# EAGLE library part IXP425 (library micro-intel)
Intel XScale® Core Source: ftp://download.intel.com/design/network/datashts/25247904.pdf
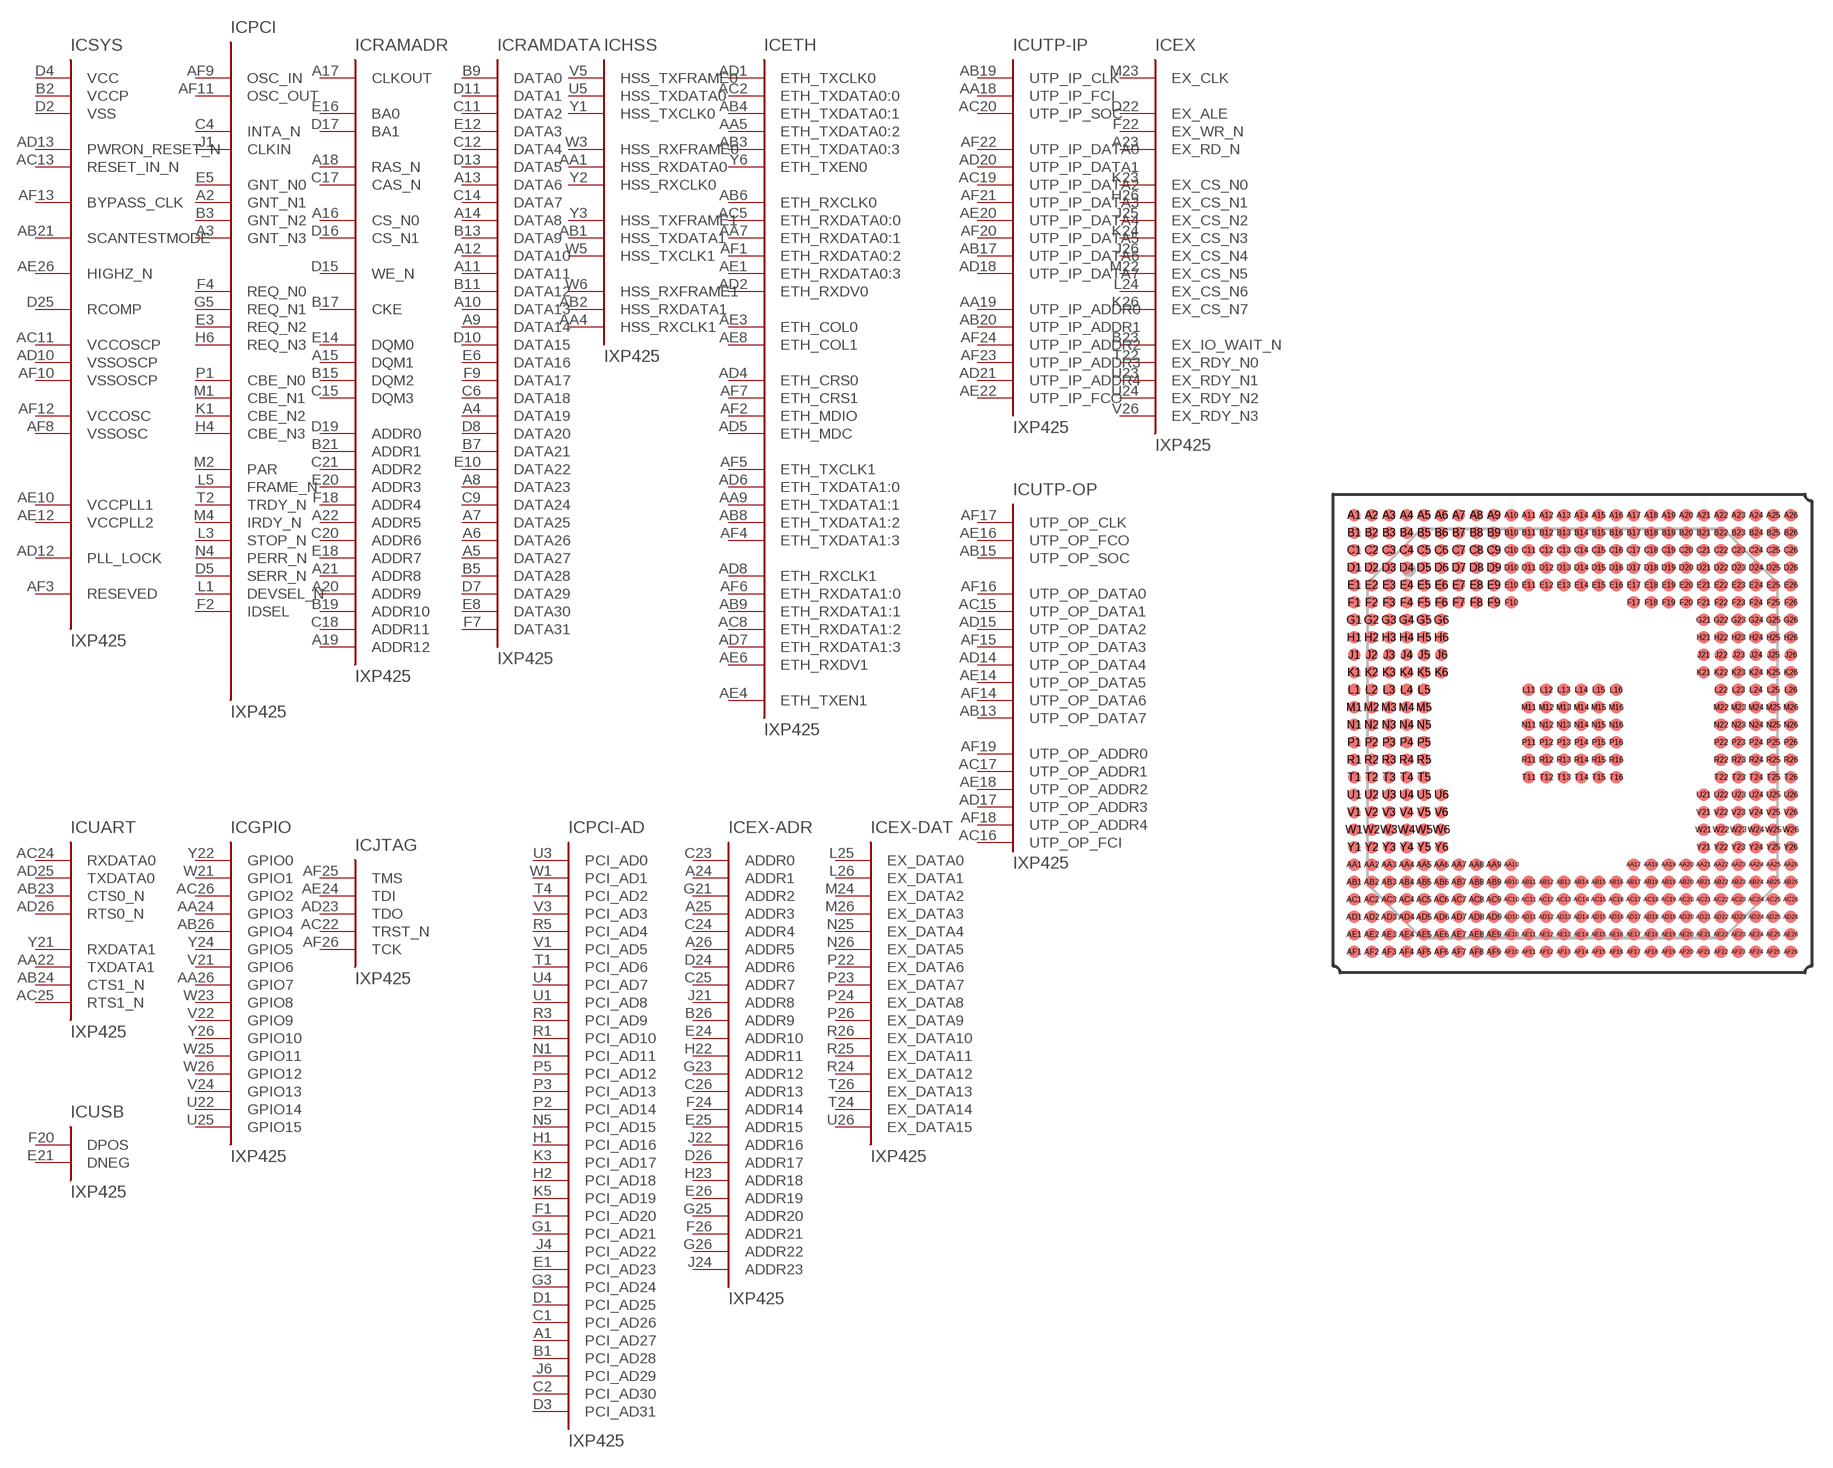
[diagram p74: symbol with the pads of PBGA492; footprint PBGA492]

Designator prefix IC; gates SYS=IXP-SYS PCI=IXP-PCI RAMADR=IXP-SDM-ADDR HSS=IXP-HSS ETH=IXP-ETH UTP-IP=IXP-UTP-IP UTP-OP=IXP-UTP-OP EX=IXP-EX UART=IXP-UART USB=IXP-USB GPIO=IXP-GPIO JTAG=IXP-JTAG PCI-AD=IXP-PCI-AD EX-ADR=IXP-EX-ADDR EX-DAT=IXP-EX-DATA RAMDATA=IXP-SDM-DATA P=IXP-PWR

## IXP425 (OC_FARNELL: unknown; OC_NEWARK: unknown)  [PBGA492]
A1  PCI-AD:PCI_AD27
A2  PCI:GNT_N1  out
A3  PCI:GNT_N3  out
A4  RAMDATA:DATA19
A5  RAMDATA:DATA27
A6  RAMDATA:DATA26
A7  RAMDATA:DATA25
A8  RAMDATA:DATA23
A9  RAMDATA:DATA14
A10  RAMDATA:DATA13
A11  RAMDATA:DATA11
A12  RAMDATA:DATA10
A13  RAMDATA:DATA6
A14  RAMDATA:DATA8
A15  RAMADR:DQM1
A16  RAMADR:CS_N0  out
A17  RAMADR:CLKOUT  out
A18  RAMADR:RAS_N  out
A19  RAMADR:ADDR12  out
A20  RAMADR:ADDR9  out
A21  RAMADR:ADDR8  out
A22  RAMADR:ADDR5  out
A23  EX:EX_RD_N  out
A24  EX-ADR:ADDR1
A25  EX-ADR:ADDR3
A26  EX-ADR:ADDR5
AA1  HSS:HSS_RXDATA0  in
AA2  P:VCCP  pwr
AA3  P:VSS  pwr
AA4  HSS:HSS_RXCLK1
AA5  ETH:ETH_TXDATA0:2  out
AA6  P:VCC  pwr
AA7  ETH:ETH_RXDATA0:1  in
AA8  P:VSS  pwr
AA9  ETH:ETH_TXDATA1:1  out
AA10  P:VCC  pwr
AA17  P:VCC  pwr
AA18  UTP-IP:UTP_IP_FCI  in
AA19  UTP-IP:UTP_IP_ADDR0  out
AA20  P:VSS  pwr
AA21  P:VCC  pwr
AA22  UART:TXDATA1  out
AA23  P:VSS  pwr
AA24  GPIO:GPIO3
AA25  P:VSS  pwr
AA26  GPIO:GPIO7
AB1  HSS:HSS_TXDATA1  out
AB2  HSS:HSS_RXDATA1  in
AB3  ETH:ETH_TXDATA0:3  out
AB4  ETH:ETH_TXDATA0:1  out
AB5  P:VSS  pwr
AB6  ETH:ETH_RXCLK0  in
AB7  P:VCCP  pwr
AB8  ETH:ETH_TXDATA1:2  out
AB9  ETH:ETH_RXDATA1:1  in
AB10  P:VCCP  pwr
AB11  P:VCCP  pwr
AB12  P:VSS  pwr
AB13  UTP-OP:UTP_OP_DATA7  out
AB14  P:VCCP  pwr
AB15  UTP-OP:UTP_OP_SOC  out
AB16  P:VSS  pwr
AB17  UTP-IP:UTP_IP_DATA6  in
AB18  P:VCCP  pwr
AB19  UTP-IP:UTP_IP_CLK  in
AB20  UTP-IP:UTP_IP_ADDR1  out
AB21  SYS:SCANTESTMODE  in
AB22  P:VCCP  pwr
AB23  UART:CTS0_N  in
AB24  UART:CTS1_N  in
AB25  P:VCCP  pwr
AB26  GPIO:GPIO4
AC1  P:VSS  pwr
AC2  ETH:ETH_TXDATA0:0  out
AC3  P:VCCP  pwr
AC4  P:VCC  pwr
AC5  ETH:ETH_RXDATA0:0  in
AC6  P:VSS  pwr
AC7  P:VCC  pwr
AC8  ETH:ETH_RXDATA1:2  in
AC9  P:VCC  pwr
AC10  P:VCC  pwr
AC11  SYS:VCCOSCP  pwr
AC12  P:VCC  pwr
AC13  SYS:RESET_IN_N  in
AC14  P:VCC  pwr
AC15  UTP-OP:UTP_OP_DATA1  out
AC16  UTP-OP:UTP_OP_FCI  in
AC17  UTP-OP:UTP_OP_ADDR1  out
AC18  P:VCC  pwr
AC19  UTP-IP:UTP_IP_DATA2  in
AC20  UTP-IP:UTP_IP_SOC  in
AC21  P:VCC  pwr
AC22  JTAG:TRST_N  in
AC23  P:VCC  pwr
AC24  UART:RXDATA0  in
AC25  UART:RTS1_N  out
AC26  GPIO:GPIO2
AD1  ETH:ETH_TXCLK0  in
AD2  ETH:ETH_RXDV0  in
AD3  P:VSS  pwr
AD4  ETH:ETH_CRS0  in
AD5  ETH:ETH_MDC  out
AD6  ETH:ETH_TXDATA1:0  out
AD7  ETH:ETH_RXDATA1:3  in
AD8  ETH:ETH_RXCLK1  in
AD9  P:VSS  pwr
AD10  SYS:VSSOSCP  pwr
AD11  P:VCCP  pwr
AD12  SYS:PLL_LOCK  out
AD13  SYS:PWRON_RESET_N  in
AD14  UTP-OP:UTP_OP_DATA4  out
AD15  UTP-OP:UTP_OP_DATA2  out
AD16  P:VSS  pwr
AD17  UTP-OP:UTP_OP_ADDR3  out
AD18  UTP-IP:UTP_IP_DATA7  in
AD19  P:VCCP  pwr
AD20  UTP-IP:UTP_IP_DATA1  in
AD21  UTP-IP:UTP_IP_ADDR4  out
AD22  P:VSS  pwr
AD23  JTAG:TDO  out
AD24  P:VSS  pwr
AD25  UART:TXDATA0  out
AD26  UART:RTS0_N  out
AE1  ETH:ETH_RXDATA0:3  in
AE2  P:VCCP  pwr
AE3  ETH:ETH_COL0
AE4  ETH:ETH_TXEN1
AE5  P:VCCP  pwr
AE6  ETH:ETH_RXDV1
AE7  P:VSS  pwr
AE8  ETH:ETH_COL1
AE9  P:VCCP  pwr
AE10  SYS:VCCPLL1  pwr
AE11  P:VSS  pwr
AE12  SYS:VCCPLL2  pwr
AE13  P:VCCP  pwr
AE14  UTP-OP:UTP_OP_DATA5  out
AE15  P:VSS  pwr
AE16  UTP-OP:UTP_OP_FCO  out
AE17  P:VCCP  pwr
AE18  UTP-OP:UTP_OP_ADDR2  out
AE19  P:VSS  pwr
AE20  UTP-IP:UTP_IP_DATA4  in
AE21  P:VCCP  pwr
AE22  UTP-IP:UTP_IP_FCO  out
AE23  P:VCCP  pwr
AE24  JTAG:TDI  in
AE25  P:VCCP  pwr
AE26  SYS:HIGHZ_N  in
AF1  ETH:ETH_RXDATA0:2  in
AF2  ETH:ETH_MDIO
AF3  SYS:RESEVED  nc
AF4  ETH:ETH_TXDATA1:3  out
AF5  ETH:ETH_TXCLK1  out
AF6  ETH:ETH_RXDATA1:0  in
AF7  ETH:ETH_CRS1  in
AF8  SYS:VSSOSC  pwr
AF9  PCI:OSC_IN  in
AF10  SYS:VSSOSCP  pwr
AF11  PCI:OSC_OUT  out
AF12  SYS:VCCOSC  pwr
AF13  SYS:BYPASS_CLK  in
AF14  UTP-OP:UTP_OP_DATA6  out
AF15  UTP-OP:UTP_OP_DATA3  out
AF16  UTP-OP:UTP_OP_DATA0  out
AF17  UTP-OP:UTP_OP_CLK  in
AF18  UTP-OP:UTP_OP_ADDR4  out
AF19  UTP-OP:UTP_OP_ADDR0  out
AF20  UTP-IP:UTP_IP_DATA5  in
AF21  UTP-IP:UTP_IP_DATA3  in
AF22  UTP-IP:UTP_IP_DATA0  in
AF23  UTP-IP:UTP_IP_ADDR3  out
AF24  UTP-IP:UTP_IP_ADDR2  out
AF25  JTAG:TMS  in
AF26  JTAG:TCK  in
B1  PCI-AD:PCI_AD28
B2  SYS:VCCP  pwr
B3  PCI:GNT_N2  out
B4  P:VCCP  pwr
B5  RAMDATA:DATA28
B6  P:VCCP  pwr
B7  RAMDATA:DATA21
B8  P:VSS  pwr
B9  RAMDATA:DATA0
B10  P:VCCP  pwr
B11  RAMDATA:DATA12
B12  P:VSS  pwr
B13  RAMDATA:DATA9
B14  P:VCCP  pwr
B15  RAMADR:DQM2
B16  P:VSS  pwr
B17  RAMADR:CKE  out
B18  P:VCCP  pwr
B19  RAMADR:ADDR10  out
B20  P:VSS  pwr
B21  RAMADR:ADDR1  out
B22  P:VCCP  pwr
B23  EX:EX_IO_WAIT_N  in
B24  P:VSS  pwr
B25  P:VCCP  pwr
B26  EX-ADR:ADDR9
C1  PCI-AD:PCI_AD26
C2  PCI-AD:PCI_AD30
C3  P:VSS  pwr
C4  PCI:INTA_N  out
C5  P:VSS  pwr
C6  RAMDATA:DATA18
C7  P:VSS  pwr
C8  P:VCCP  pwr
C9  RAMDATA:DATA24
C10  P:VSS  pwr
C11  RAMDATA:DATA2
C12  RAMDATA:DATA4
C13  P:VSS  pwr
C14  RAMDATA:DATA7
C15  RAMADR:DQM3
C16  P:VCCP  pwr
C17  RAMADR:CAS_N  out
C18  RAMADR:ADDR11  out
C19  P:VSS  pwr
C20  RAMADR:ADDR6  out
C21  RAMADR:ADDR2  out
C22  P:VSS  pwr
C23  EX-ADR:ADDR0
C24  EX-ADR:ADDR4
C25  EX-ADR:ADDR7
C26  EX-ADR:ADDR13
D1  PCI-AD:PCI_AD25
D2  SYS:VSS  pwr
D3  PCI-AD:PCI_AD31
D4  SYS:VCC  pwr
D5  PCI:SERR_N
D6  P:VCC  pwr
D7  RAMDATA:DATA29
D8  RAMDATA:DATA20
D9  P:VCC  pwr
D10  RAMDATA:DATA15
D11  RAMDATA:DATA1
D12  P:VCC  pwr
D13  RAMDATA:DATA5
D14  P:VCC  pwr
D15  RAMADR:WE_N  out
D16  RAMADR:CS_N1  out
D17  RAMADR:BA1  out
D18  P:VCC  pwr
D19  RAMADR:ADDR0  out
D20  P:VSS  pwr
D21  P:VCC  pwr
D22  EX:EX_ALE  out
D23  P:VCC  pwr
D24  EX-ADR:ADDR6
D25  SYS:RCOMP  in
D26  EX-ADR:ADDR17
E1  PCI-AD:PCI_AD23
E2  P:VCCP  pwr
E3  PCI:REQ_N2  in
E4  P:VSS  pwr
E5  PCI:GNT_N0
E6  RAMDATA:DATA16
E7  P:VCCP  pwr
E8  RAMDATA:DATA30
E9  P:VSS  pwr
E10  RAMDATA:DATA22
E11  P:VCCP  pwr
E12  RAMDATA:DATA3
E13  P:VSS  pwr
E14  RAMADR:DQM0
E15  P:VCCP  pwr
E16  RAMADR:BA0  out
E17  P:VSS  pwr
E18  RAMADR:ADDR7  out
E19  P:VCCP  pwr
E20  RAMADR:ADDR3  out
E21  USB:DNEG
E22  P:VCCP  pwr
E23  P:VSS  pwr
E24  EX-ADR:ADDR10
E25  EX-ADR:ADDR15
E26  EX-ADR:ADDR19
F1  PCI-AD:PCI_AD20
F2  PCI:IDSEL  in
F3  P:VCC  pwr
F4  PCI:REQ_N0
F5  P:VCCP  pwr
F6  P:VCC  pwr
F7  RAMDATA:DATA31
F8  P:VSS  pwr
F9  RAMDATA:DATA17
F10  P:VCC  pwr
F17  P:VCC  pwr
F18  RAMADR:ADDR4  out
F19  P:VSS  pwr
F20  USB:DPOS
F21  P:VCC  pwr
F22  EX:EX_WR_N  out
F23  P:VCC  pwr
F24  EX-ADR:ADDR14
F25  P:VCCP  pwr
F26  EX-ADR:ADDR21
G1  PCI-AD:PCI_AD21
G2  P:VCCP  pwr
G3  PCI-AD:PCI_AD24
G4  P:VSS  pwr
G5  PCI:REQ_N1  in
G6  P:VSS  pwr
G21  EX-ADR:ADDR2
G22  P:VSS  pwr
G23  EX-ADR:ADDR12
G24  P:VSS  pwr
G25  EX-ADR:ADDR20
G26  EX-ADR:ADDR22
H1  PCI-AD:PCI_AD16
H2  PCI-AD:PCI_AD18
H3  P:VCC  pwr
H4  PCI:CBE_N3
H5  P:VCC  pwr
H6  PCI:REQ_N3  in
H21  P:VSS  pwr
H22  EX-ADR:ADDR11
H23  EX-ADR:ADDR18
H24  P:VCCP  pwr
H25  P:VSS  pwr
H26  EX:EX_CS_N1  out
J1  PCI:CLKIN  in
J2  P:VCCP  pwr
J3  P:VSS  pwr
J4  PCI-AD:PCI_AD22
J5  P:VSS  pwr
J6  PCI-AD:PCI_AD29
J21  EX-ADR:ADDR8
J22  EX-ADR:ADDR16
J23  P:VCC  pwr
J24  EX-ADR:ADDR23
J25  EX:EX_CS_N2  out
J26  EX:EX_CS_N4  out
K1  PCI:CBE_N2
K2  P:VSS  pwr
K3  PCI-AD:PCI_AD17
K4  P:VCCP  pwr
K5  PCI-AD:PCI_AD19
K6  P:VCC  pwr
K21  P:VCC  pwr
K22  P:VSS  pwr
K23  EX:EX_CS_N0  out
K24  EX:EX_CS_N3  out
K25  P:VCCP  pwr
K26  EX:EX_CS_N7  out
L1  PCI:DEVSEL_N
L2  P:VCCP  pwr
L3  PCI:STOP_N
L4  P:VCC  pwr
L5  PCI:FRAME_N
L11  P:VSS  pwr
L12  P:VSS  pwr
L13  P:VSS  pwr
L14  P:VSS  pwr
L15  P:VSS  pwr
L16  P:VSS  pwr
L22  P:VCCP  pwr
L23  P:VCC  pwr
L24  EX:EX_CS_N6  out
L25  EX-DAT:EX_DATA0
L26  EX-DAT:EX_DATA1
M1  PCI:CBE_N1
M2  PCI:PAR
M3  P:VSS  pwr
M4  PCI:IRDY_N
M5  P:VCCP  pwr
M11  P:VSS  pwr
M12  P:VSS  pwr
M13  P:VSS  pwr
M14  P:VSS  pwr
M15  P:VSS  pwr
M16  P:VSS  pwr
M22  EX:EX_CS_N5  out
M23  EX:EX_CLK  in
M24  EX-DAT:EX_DATA2
M25  P:VSS  pwr
M26  EX-DAT:EX_DATA3
N1  PCI-AD:PCI_AD11
N2  P:VCCP  pwr
N3  P:VCC  pwr
N4  PCI:PERR_N
N5  PCI-AD:PCI_AD15
N11  P:VSS  pwr
N12  P:VSS  pwr
N13  P:VSS  pwr
N14  P:VSS  pwr
N15  P:VSS  pwr
N16  P:VSS  pwr
N22  P:VCC  pwr
N23  P:VSS  pwr
N24  P:VCC  pwr
N25  EX-DAT:EX_DATA4
N26  EX-DAT:EX_DATA5
P1  PCI:CBE_N0
P2  PCI-AD:PCI_AD14
P3  PCI-AD:PCI_AD13
P4  P:VSS  pwr
P5  PCI-AD:PCI_AD12
P11  P:VSS  pwr
P12  P:VSS  pwr
P13  P:VSS  pwr
P14  P:VSS  pwr
P15  P:VSS  pwr
P16  P:VSS  pwr
P22  EX-DAT:EX_DATA6
P23  EX-DAT:EX_DATA7
P24  EX-DAT:EX_DATA8
P25  P:VCCP  pwr
P26  EX-DAT:EX_DATA9
R1  PCI-AD:PCI_AD10
R2  P:VSS  pwr
R3  PCI-AD:PCI_AD9
R4  P:VCC  pwr
R5  PCI-AD:PCI_AD4
R11  P:VSS  pwr
R12  P:VSS  pwr
R13  P:VSS  pwr
R14  P:VSS  pwr
R15  P:VSS  pwr
R16  P:VSS  pwr
R22  P:VCCP  pwr
R23  P:VCC  pwr
R24  EX-DAT:EX_DATA12
R25  EX-DAT:EX_DATA11
R26  EX-DAT:EX_DATA10
T1  PCI-AD:PCI_AD6
T2  PCI:TRDY_N
T3  P:VSS  pwr
T4  PCI-AD:PCI_AD2
T5  P:VCCP  pwr
T11  P:VSS  pwr
T12  P:VSS  pwr
T13  P:VSS  pwr
T14  P:VSS  pwr
T15  P:VSS  pwr
T16  P:VSS  pwr
T22  EX:EX_RDY_N0  in
T23  P:VSS  pwr
T24  EX-DAT:EX_DATA14
T25  P:VSS  pwr
T26  EX-DAT:EX_DATA13
U1  PCI-AD:PCI_AD8
U2  P:VCCP  pwr
U3  PCI-AD:PCI_AD0
U4  PCI-AD:PCI_AD7
U5  HSS:HSS_TXDATA0  out
U6  P:VCC  pwr
U21  P:VCC  pwr
U22  GPIO:GPIO14
U23  EX:EX_RDY_N1  in
U24  EX:EX_RDY_N2  in
U25  GPIO:GPIO15
U26  EX-DAT:EX_DATA15
V1  PCI-AD:PCI_AD5
V2  P:VSS  pwr
V3  PCI-AD:PCI_AD3
V4  P:VCC  pwr
V5  HSS:HSS_TXFRAME0
V6  P:VSS  pwr
V21  GPIO:GPIO6
V22  GPIO:GPIO9
V23  P:VCC  pwr
V24  GPIO:GPIO13
V25  P:VCCP  pwr
V26  EX:EX_RDY_N3  in
W1  PCI-AD:PCI_AD1
W2  P:VCCP  pwr
W3  HSS:HSS_RXFRAME0
W4  P:VSS  pwr
W5  HSS:HSS_TXCLK1
W6  HSS:HSS_RXFRAME1
W21  GPIO:GPIO1
W22  P:VCCP  pwr
W23  GPIO:GPIO8
W24  P:VSS  pwr
W25  GPIO:GPIO11
W26  GPIO:GPIO12
Y1  HSS:HSS_TXCLK0
Y2  HSS:HSS_RXCLK0
Y3  HSS:HSS_TXFRAME1
Y4  P:VCC  pwr
Y5  P:VCCP  pwr
Y6  ETH:ETH_TXEN0  out
Y21  UART:RXDATA1  in
Y22  GPIO:GPIO0
Y23  P:VCC  pwr
Y24  GPIO:GPIO5
Y25  P:VCCP  pwr
Y26  GPIO:GPIO10

## Footprint PBGA492 (pad centres in mm)
492-Pin Lead PBGA (plastic ball grid array) Source: ftp://download.intel.com/design/network/datashts/25247904.pdf
smd 0.9 x 0.9: A1 -15.875,15.875; A2 -14.605,15.875; A3 -13.335,15.875; A4 -12.065,15.875; A5 -10.795,15.875; A6 -9.525,15.875; A7 -8.255,15.875; A8 -6.985,15.875; A9 -5.715,15.875; A10 -4.445,15.875; A11 -3.175,15.875; A12 -1.905,15.875; A13 -0.635,15.875; A14 0.635,15.875; A15 1.905,15.875; A16 3.175,15.875; A17 4.445,15.875; A18 5.715,15.875; A19 6.985,15.875; A20 8.255,15.875; A21 9.525,15.875; A22 10.795,15.875; A23 12.065,15.875; A24 13.335,15.875; A25 14.605,15.875; A26 15.875,15.875; AA1 -15.875,-9.525; AA2 -14.605,-9.525; AA3 -13.335,-9.525; AA4 -12.065,-9.525; AA5 -10.795,-9.525; AA6 -9.525,-9.525; AA7 -8.255,-9.525; AA8 -6.985,-9.525; AA9 -5.715,-9.525; AA10 -4.445,-9.525; AA17 4.445,-9.525; AA18 5.715,-9.525; AA19 6.985,-9.525; AA20 8.255,-9.525; AA21 9.525,-9.525; AA22 10.795,-9.525; AA23 12.065,-9.525; AA24 13.335,-9.525; AA25 14.605,-9.525; AA26 15.875,-9.525; AB1 -15.875,-10.795; AB2 -14.605,-10.795; AB3 -13.335,-10.795; AB4 -12.065,-10.795; AB5 -10.795,-10.795; AB6 -9.525,-10.795; AB7 -8.255,-10.795; AB8 -6.985,-10.795; AB9 -5.715,-10.795; AB10 -4.445,-10.795; AB11 -3.175,-10.795; AB12 -1.905,-10.795; AB13 -0.635,-10.795; AB14 0.635,-10.795; AB15 1.905,-10.795; AB16 3.175,-10.795; AB17 4.445,-10.795; AB18 5.715,-10.795; AB19 6.985,-10.795; AB20 8.255,-10.795; AB21 9.525,-10.795; AB22 10.795,-10.795; AB23 12.065,-10.795; AB24 13.335,-10.795; AB25 14.605,-10.795; AB26 15.875,-10.795; AC1 -15.875,-12.065; AC2 -14.605,-12.065; AC3 -13.335,-12.065; AC4 -12.065,-12.065; AC5 -10.795,-12.065; AC6 -9.525,-12.065; AC7 -8.255,-12.065; AC8 -6.985,-12.065; AC9 -5.715,-12.065; AC10 -4.445,-12.065; AC11 -3.175,-12.065; AC12 -1.905,-12.065; AC13 -0.635,-12.065; AC14 0.635,-12.065; AC15 1.905,-12.065; AC16 3.175,-12.065; AC17 4.445,-12.065; AC18 5.715,-12.065; AC19 6.985,-12.065; AC20 8.255,-12.065; AC21 9.525,-12.065; AC22 10.795,-12.065; AC23 12.065,-12.065; AC24 13.335,-12.065; AC25 14.605,-12.065; AC26 15.875,-12.065; AD1 -15.875,-13.335; AD2 -14.605,-13.335; AD3 -13.335,-13.335; AD4 -12.065,-13.335; AD5 -10.795,-13.335; AD6 -9.525,-13.335; AD7 -8.255,-13.335; AD8 -6.985,-13.335; AD9 -5.715,-13.335; AD10 -4.445,-13.335; AD11 -3.175,-13.335; AD12 -1.905,-13.335; AD13 -0.635,-13.335; AD14 0.635,-13.335; AD15 1.905,-13.335; AD16 3.175,-13.335; AD17 4.445,-13.335; AD18 5.715,-13.335; AD19 6.985,-13.335; AD20 8.255,-13.335; AD21 9.525,-13.335; AD22 10.795,-13.335; AD23 12.065,-13.335; AD24 13.335,-13.335; AD25 14.605,-13.335; AD26 15.875,-13.335; AE1 -15.875,-14.605; AE2 -14.605,-14.605; AE3 -13.335,-14.605; AE4 -12.065,-14.605; AE5 -10.795,-14.605; AE6 -9.525,-14.605; AE7 -8.255,-14.605; AE8 -6.985,-14.605; AE9 -5.715,-14.605; AE10 -4.445,-14.605; AE11 -3.175,-14.605; AE12 -1.905,-14.605; AE13 -0.635,-14.605; AE14 0.635,-14.605; AE15 1.905,-14.605; AE16 3.175,-14.605; AE17 4.445,-14.605; AE18 5.715,-14.605; AE19 6.985,-14.605; AE20 8.255,-14.605; AE21 9.525,-14.605; AE22 10.795,-14.605; AE23 12.065,-14.605; AE24 13.335,-14.605; AE25 14.605,-14.605; AE26 15.875,-14.605; AF1 -15.875,-15.875; AF2 -14.605,-15.875; AF3 -13.335,-15.875; AF4 -12.065,-15.875; AF5 -10.795,-15.875; AF6 -9.525,-15.875; AF7 -8.255,-15.875; AF8 -6.985,-15.875; AF9 -5.715,-15.875; AF10 -4.445,-15.875; AF11 -3.175,-15.875; AF12 -1.905,-15.875; AF13 -0.635,-15.875; AF14 0.635,-15.875; AF15 1.905,-15.875; AF16 3.175,-15.875; AF17 4.445,-15.875; AF18 5.715,-15.875; AF19 6.985,-15.875; AF20 8.255,-15.875; AF21 9.525,-15.875; AF22 10.795,-15.875; AF23 12.065,-15.875; AF24 13.335,-15.875; AF25 14.605,-15.875; AF26 15.875,-15.875; B1 -15.875,14.605; B2 -14.605,14.605; B3 -13.335,14.605; B4 -12.065,14.605; B5 -10.795,14.605; B6 -9.525,14.605; B7 -8.255,14.605; B8 -6.985,14.605; B9 -5.715,14.605; B10 -4.445,14.605; B11 -3.175,14.605; B12 -1.905,14.605; B13 -0.635,14.605; B14 0.635,14.605; B15 1.905,14.605; B16 3.175,14.605; B17 4.445,14.605; B18 5.715,14.605; B19 6.985,14.605; B20 8.255,14.605; B21 9.525,14.605; B22 10.795,14.605; B23 12.065,14.605; B24 13.335,14.605; B25 14.605,14.605; B26 15.875,14.605; C1 -15.875,13.335; C2 -14.605,13.335; C3 -13.335,13.335; C4 -12.065,13.335; C5 -10.795,13.335; C6 -9.525,13.335; C7 -8.255,13.335; C8 -6.985,13.335; C9 -5.715,13.335; C10 -4.445,13.335; C11 -3.175,13.335; C12 -1.905,13.335; C13 -0.635,13.335; C14 0.635,13.335; C15 1.905,13.335; C16 3.175,13.335; C17 4.445,13.335; C18 5.715,13.335; C19 6.985,13.335; C20 8.255,13.335; C21 9.525,13.335; C22 10.795,13.335; C23 12.065,13.335; C24 13.335,13.335; C25 14.605,13.335; C26 15.875,13.335; D1 -15.875,12.065; D2 -14.605,12.065; D3 -13.335,12.065; D4 -12.065,12.065; D5 -10.795,12.065; D6 -9.525,12.065; D7 -8.255,12.065; D8 -6.985,12.065; D9 -5.715,12.065; D10 -4.445,12.065; D11 -3.175,12.065; D12 -1.905,12.065; D13 -0.635,12.065; D14 0.635,12.065; D15 1.905,12.065; D16 3.175,12.065; D17 4.445,12.065; D18 5.715,12.065; D19 6.985,12.065; D20 8.255,12.065; D21 9.525,12.065; D22 10.795,12.065; D23 12.065,12.065; D24 13.335,12.065; D25 14.605,12.065; D26 15.875,12.065; E1 -15.875,10.795; E2 -14.605,10.795; E3 -13.335,10.795; E4 -12.065,10.795; E5 -10.795,10.795; E6 -9.525,10.795; E7 -8.255,10.795; E8 -6.985,10.795; E9 -5.715,10.795; E10 -4.445,10.795; E11 -3.175,10.795; E12 -1.905,10.795; E13 -0.635,10.795; E14 0.635,10.795; E15 1.905,10.795; E16 3.175,10.795; E17 4.445,10.795; E18 5.715,10.795; E19 6.985,10.795; E20 8.255,10.795; E21 9.525,10.795; E22 10.795,10.795; E23 12.065,10.795; E24 13.335,10.795; E25 14.605,10.795; E26 15.875,10.795; F1 -15.875,9.525; F2 -14.605,9.525; F3 -13.335,9.525; F4 -12.065,9.525; F5 -10.795,9.525; F6 -9.525,9.525; F7 -8.255,9.525; F8 -6.985,9.525; F9 -5.715,9.525; F10 -4.445,9.525; F17 4.445,9.525; F18 5.715,9.525; F19 6.985,9.525; F20 8.255,9.525; F21 9.525,9.525; F22 10.795,9.525; F23 12.065,9.525; F24 13.335,9.525; F25 14.605,9.525; F26 15.875,9.525; G1 -15.875,8.255; G2 -14.605,8.255; G3 -13.335,8.255; G4 -12.065,8.255; G5 -10.795,8.255; G6 -9.525,8.255; G21 9.525,8.255; G22 10.795,8.255; G23 12.065,8.255; G24 13.335,8.255; G25 14.605,8.255; G26 15.875,8.255; H1 -15.875,6.985; H2 -14.605,6.985; H3 -13.335,6.985; H4 -12.065,6.985; H5 -10.795,6.985; H6 -9.525,6.985; H21 9.525,6.985; H22 10.795,6.985; H23 12.065,6.985; H24 13.335,6.985; H25 14.605,6.985; H26 15.875,6.985; J1 -15.875,5.715; J2 -14.605,5.715; J3 -13.335,5.715; J4 -12.065,5.715; J5 -10.795,5.715; J6 -9.525,5.715; J21 9.525,5.715; J22 10.795,5.715; J23 12.065,5.715; J24 13.335,5.715; J25 14.605,5.715; J26 15.875,5.715; K1 -15.875,4.445; K2 -14.605,4.445; K3 -13.335,4.445; K4 -12.065,4.445; K5 -10.795,4.445; K6 -9.525,4.445; K21 9.525,4.445; K22 10.795,4.445; K23 12.065,4.445; K24 13.335,4.445; K25 14.605,4.445; K26 15.875,4.445; L1 -15.875,3.175; L2 -14.605,3.175; L3 -13.335,3.175; L4 -12.065,3.175; L5 -10.795,3.175; L11 -3.175,3.175; L12 -1.905,3.175; L13 -0.635,3.175; L14 0.635,3.175; L15 1.905,3.175; L16 3.175,3.175; L22 10.795,3.175; L23 12.065,3.175; L24 13.335,3.175; L25 14.605,3.175; L26 15.875,3.175; M1 -15.875,1.905; M2 -14.605,1.905; M3 -13.335,1.905; M4 -12.065,1.905; M5 -10.795,1.905; M11 -3.175,1.905; M12 -1.905,1.905; M13 -0.635,1.905; M14 0.635,1.905; M15 1.905,1.905; M16 3.175,1.905; M22 10.795,1.905; M23 12.065,1.905; M24 13.335,1.905; M25 14.605,1.905; M26 15.875,1.905; N1 -15.875,0.635; N2 -14.605,0.635; N3 -13.335,0.635; N4 -12.065,0.635; N5 -10.795,0.635; N11 -3.175,0.635; N12 -1.905,0.635; N13 -0.635,0.635; N14 0.635,0.635; N15 1.905,0.635; N16 3.175,0.635; N22 10.795,0.635; N23 12.065,0.635; N24 13.335,0.635; N25 14.605,0.635; N26 15.875,0.635; P1 -15.875,-0.635; P2 -14.605,-0.635; P3 -13.335,-0.635; P4 -12.065,-0.635; P5 -10.795,-0.635; P11 -3.175,-0.635; P12 -1.905,-0.635; P13 -0.635,-0.635; P14 0.635,-0.635; P15 1.905,-0.635; P16 3.175,-0.635; P22 10.795,-0.635; P23 12.065,-0.635; P24 13.335,-0.635; P25 14.605,-0.635; P26 15.875,-0.635; R1 -15.875,-1.905; R2 -14.605,-1.905; R3 -13.335,-1.905; R4 -12.065,-1.905; R5 -10.795,-1.905; R11 -3.175,-1.905; R12 -1.905,-1.905; R13 -0.635,-1.905; R14 0.635,-1.905; R15 1.905,-1.905; R16 3.175,-1.905; R22 10.795,-1.905; R23 12.065,-1.905; R24 13.335,-1.905; R25 14.605,-1.905; R26 15.875,-1.905; T1 -15.875,-3.175; T2 -14.605,-3.175; T3 -13.335,-3.175; T4 -12.065,-3.175; T5 -10.795,-3.175; T11 -3.175,-3.175; T12 -1.905,-3.175; T13 -0.635,-3.175; T14 0.635,-3.175; T15 1.905,-3.175; T16 3.175,-3.175; T22 10.795,-3.175; T23 12.065,-3.175; T24 13.335,-3.175; T25 14.605,-3.175; T26 15.875,-3.175; U1 -15.875,-4.445; U2 -14.605,-4.445; U3 -13.335,-4.445; U4 -12.065,-4.445; U5 -10.795,-4.445; U6 -9.525,-4.445; U21 9.525,-4.445; U22 10.795,-4.445; U23 12.065,-4.445; U24 13.335,-4.445; U25 14.605,-4.445; U26 15.875,-4.445; V1 -15.875,-5.715; V2 -14.605,-5.715; V3 -13.335,-5.715; V4 -12.065,-5.715; V5 -10.795,-5.715; V6 -9.525,-5.715; V21 9.525,-5.715; V22 10.795,-5.715; V23 12.065,-5.715; V24 13.335,-5.715; V25 14.605,-5.715; V26 15.875,-5.715; W1 -15.875,-6.985; W2 -14.605,-6.985; W3 -13.335,-6.985; W4 -12.065,-6.985; W5 -10.795,-6.985; W6 -9.525,-6.985; W21 9.525,-6.985; W22 10.795,-6.985; W23 12.065,-6.985; W24 13.335,-6.985; W25 14.605,-6.985; W26 15.875,-6.985; Y1 -15.875,-8.255; Y2 -14.605,-8.255; Y3 -13.335,-8.255; Y4 -12.065,-8.255; Y5 -10.795,-8.255; Y6 -9.525,-8.255; Y21 9.525,-8.255; Y22 10.795,-8.255; Y23 12.065,-8.255; Y24 13.335,-8.255; Y25 14.605,-8.255; Y26 15.875,-8.255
